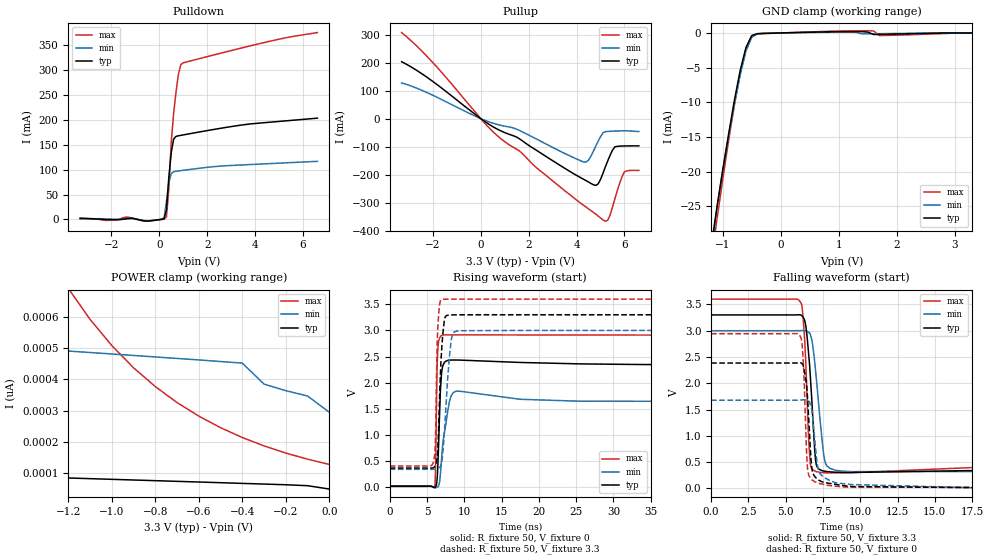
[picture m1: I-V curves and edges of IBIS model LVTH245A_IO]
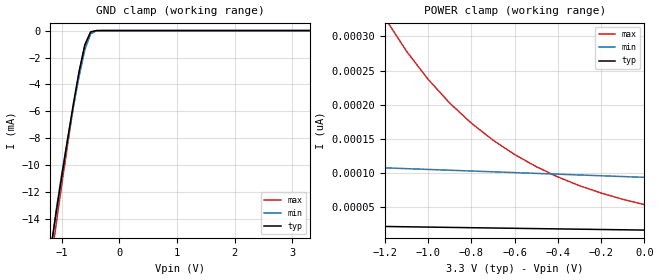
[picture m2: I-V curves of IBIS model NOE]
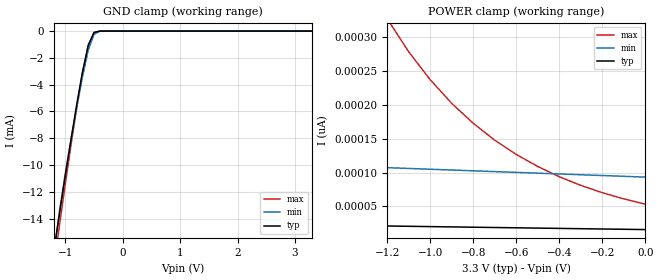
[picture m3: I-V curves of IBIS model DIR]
|   TEXAS INSTRUMENTS INCORPORATED
|   Standard Linear and Logic
|   IBIS Model of SN54LVTH245A
|   3.3V ABT OCTAL BUS  TRANSCEIVERS WITH 3-STATE OUTPUT
| This file contains package information for the following:
|   CFP 20-pin (W) package as [Component] LVTH245A_W
[IBIS Ver]   2.1
[Comment char]   |_char
[File Name]   sn54lvth245aw.ibs
[File Rev]   1.0
[Date]   06-13-2000
[Source]   Data created from HSPICE simulations at TI ,SLL.
[Notes]   The following is an IBIS list for LVTH245A.
   - All test data contained in this file are derived from hspice
   (tm) simulations.
   - - This file may be incomplete or may not be fully compliant
   with the IBIS specification. It will be replaced with a
   version that is IBIS Revision 3.2 compliant and is complete
   and accurate. Please email all questions and comments to
   sllibis@ti.com.
|   -For Questions or Comments please mailto:sllibis@ti.com
|  [Disclaimer]
|*   Property of Texas Instruments Incorporated.  Unauthorized   *
|*   reproduction and/or distribution is strictly prohibited.   *
|*   This product is protected under copyright law.   *
|*   Created 1995, (C) Copyright 1995, Texas Instruments Inc.,   *
|*   All Rights Reserved   *
|*   UNLESS THERE IS A SIGNED, WRITTEN AGREEMENT TO THE   *
|*   CONTRARY, TEXAS INSTRUMENTS ("TI") IS PROVIDING THE SPICE   *
|*   MODELS "AS IS" AND WITHOUT ANY WARRANTY, EXPRESSED OR   *
|*   IMPLIED.  TI assumes no liability for:   *
|*   1) the accuracy of the IBIS models provided to your   *
|*   company;   *
|*   2) the proper functioning of these IBIS models in your   *
|*   design or for any resulting applications; or   *
|*   3) infringement of patents, copyrights or intellectual   *
|*   property rights resulting from your use of these   *
|*   IBIS models.   *
|*   TI provides IBIS Models as a service to our customers.   *
|*   You and your company shall not distribute, sell or give   *
|*   these models to anyone else without prior written   *
|*   permission from TI.   *
|*   TI reserves the right to make changes to our products or   *
|*   to discontinue any semiconductor product or service   *
|*   without notice, and advises our customers to obtain the   *
|*   latest version of relevant information to verify, before   *
|*   placing orders, that the information being relied on is   *
|*   current.   *
|*   Please be aware that your receipt and use of the IBIS   *
|*   information provided shall serve as acceptance of these   *
|*   terms and conditions.  If you do not accept these terms,   *
|*   you should return or destroy the IBIS models and any   *
|*   other accompanying information immediately.   *
[Component]   LVTH245A_W
[manufacturer]   Texas   Instruments,   Inc.
[Package]
|   typ   min   max
R_pkg   0.134   0.093   0.180
L_pkg   6.136e-9   4.282e-9   8.371e-9
C_pkg   1.657e-12   1.224e-12   2.253e-12
[Pin]   signal_name  model_name   R_pin   L_pin   C_pin
1   DIR   DIR   0.161   8.173e-9   2.244e-12
2   A1   LVTH245A_IO   0.163   7.152e-9   2.034e-12
3   A2   LVTH245A_IO   0.154   6.346e-9   1.604e-12
4   A3   LVTH245A_IO   0.093   4.737e-9   1.272e-12
5   A4   LVTH245A_IO   0.097   4.297e-9   1.227e-12
6   A5   LVTH245A_IO   0.096   4.289e-9   1.226e-12
7   A6   LVTH245A_IO   0.093   4.759e-9   1.269e-12
8   A7   LVTH245A_IO   0.143   6.181e-9   1.554e-12
9   A8   LVTH245A_IO   0.164   7.085e-9   1.905e-12
10   GND   GND   0.175   8.294e-9   2.233e-12
11   B8   LVTH245A_IO   0.180   8.371e-9   2.239e-12
12   B7   LVTH245A_IO   0.155   7.195e-9   1.934e-12
13   B6   LVTH245A_IO   0.154   6.339e-9   1.581e-12
14   B5   LVTH245A_IO   0.096   4.872e-9   1.281e-12
15   B4   LVTH245A_IO   0.097   4.338e-9   1.233e-12
16   B3   LVTH245A_IO   0.097   4.282e-9   1.224e-12
17   B2   LVTH245A_IO   0.093   4.726e-9   1.262e-12
18   B1   LVTH245A_IO   0.143   6.164e-9   1.571e-12
19   NOE   NOE   0.159   6.938e-9   2.001e-12
20   VCC   POWER   0.166   8.186e-9   2.253e-12
| Models and submodels in the file (3): LVTH245A_IO (I/O), NOE (Input), DIR (Input)
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|   Model LVTH245A  I/O
[Model]   LVTH245A_IO
|Signals
Model_type  I/O
Polarity   Non-Inverting
Enable   Active-Low
Vinl = 0.8V
Vinh = 2.0V
Vmeas= 1.5V
Cref = 50pf
Rref = 500
Vref = 0V
| variable   typ   min   max
C_comp   9p   NA   NA
[Temperature Range]   50   100   0
[Voltage range]   3.3   3   3.6
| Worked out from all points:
|   slope of the pulldown table from 0 to 0.495 V, typ, clamps not added: 3.74 ohm
|   slope of the pullup table from 0 to 0.495 V, typ, clamps not added: 17.5 ohm
|   GND clamp passes 1 mA (typ) near -0.54 V on its own axis
|   rising waveform, R_fixture 50, V_fixture 0: 20-80 % time 334ps typ, 787ps min, 187ps max; typ from 0.015 V to 2.34 V
|   falling waveform, R_fixture 50, V_fixture 3.3: 20-80 % time 407ps typ, 539ps min, 282ps max; typ from 3.3 V to 0.361 V
|   rising waveform, R_fixture 50, V_fixture 3.3: 20-80 % time 487ps typ, 748ps min, 267ps max; typ from 0.363 V to 3.3 V
|   falling waveform, R_fixture 50, V_fixture 0: 20-80 % time 301ps typ, 395ps min, 226ps max; typ from 2.38 V to 0.015 V
|Process range|   weak   strong
[Pullup]
|   50C:3.3V:   100C:3V:weak   0C:3.6V:strong
|   Voltage   I(typ)   I(min)   I(max)
-3.3V     203.1mA    127.3mA    307.1mA
-2V       132.7mA    83.36mA    200.3mA
500mV     -28.53mA   -16.16mA   -45.85mA
1.5V      -66.22mA   -37.93mA   -109.4mA
4.3V      -217.1mA   -155.1mA   -310.2mA
4.5V      -226.5mA   -148.4mA   -322.3mA
4.8V      -238.8mA   -98.67mA   -341.2mA
5.2V      -173.2mA   -46.97mA   -366.8mA
5.4V      -131.2mA   -45.38mA   -344.5mA
5.6V      -101.1mA   -44.62mA   -286.1mA
6V        -97.81mA   -43.69mA   -190.1mA
6.6V      -97.49mA   -46.24mA   -185.2mA
[Pulldown]
|   50C:3.3V:   100C:3V:weak   0C:3.6V:strong
|   Voltage   I(typ)   I(min)   I(max)
-3.3V     2.372mA    1.132mA    2.209mA
100mV     237.9uA    350.5uA    100.7uA
200mV     1.235mA    3.577mA    847.1uA
300mV     19.22mA    35.89mA    5.175mA
400mV     84.98mA    73.59mA    61.36mA
500mV     134.2mA    92.25mA    155.8mA
600mV     161.2mA    95.76mA    213.1mA
700mV     166.6mA    96.57mA    256.3mA
800mV     167.8mA    97.24mA    291.1mA
900mV     168.7mA    97.89mA    310.7mA
3.6V      190.4mA    109.7mA    345.9mA
6.6V      203.2mA    116.6mA    374.8mA
[GND Clamp]
|   50C:3.3V:   100C:3V:weak   0C:3.6V:strong
|   Voltage   I(typ)   I(min)   I(max)
-3.3V     -626.4mA   -591.3mA   -680.6mA
-1.2V     -30.81mA   -32.23mA   -32.92mA
-1.1V     -25.16mA   -25.2mA    -26.88mA
-900mV    -14.66mA   -14.89mA   -15.59mA
-700mV    -5.437mA   -6.128mA   -5.899mA
-600mV    -2.11mA    -2.619mA   -2.27mA
-500mV    -382.9uA   -616.2uA   -399.1uA
-200mV    -45.64uA   -31.21uA   -65.88uA
1.4V      189.6uA    -126.3uA   320.1uA
1.6V      -220.2uA   -114.9uA   285.4uA
1.7V      -211.2uA   -105.7uA   -367.5uA
3.3V      49.01pA    384.5pA    -3.178nA
[POWER Clamp]
|   50C:3.3V:   100C:3V:weak   0C:3.6V:strong
|   Voltage   I(typ)   I(min)   I(max)
-3.3V     132.6pA    589.3pA    21.93nA
-1.2V     84.38pA    490.2pA    690.3pA
-1.1V     82.21pA    485.5pA    591.4pA
-1V       80.06pA    480.8pA    507.7pA
-900mV    77.9pA     476.1pA    436.7pA
-800mV    75.76pA    471.3pA    376.5pA
-700mV    73.62pA    466.6pA    325.5pA
-600mV    71.47pA    461.9pA    282.1pA
-400mV    67.05pA    451.6pA    213.8pA
-300mV    64.88pA    384.5pA    186.9pA
-100mV    59.71pA    346.4pA    144.5pA
0V        49.01pA    294.5pA    127.6pA
[ramp]
| variable   typ   min   max
dV/dt_r   1.4680E+00/3.6232E-10  1.1128E+00/9.3641E-10  1.7543E+00/1.8433E-10
dV/dt_f   1.8000E+00/4.1355E-10  1.6130E+00/5.4301E-10  1.9843E+00/2.8338E-10
[Rising Waveform]
R_fixture = 50
V_fixture = 0
V_fixture_min =0
V_fixture_max = 0
L_fixture = 0nH
C_fixture = 0pF
|   50C:3.3V:   100C:3V:weak   0C:3.6V:strong
|   Time   V(typ)   V(min)   V(max)
0s        14.92mV    10.12mV    20.87mV
6ns       -13.42mV   -12.8mV    854.9uV
6.15ns    5.5mV      -16.5mV    391.4mV
6.35ns    142.1mV    -4.054mV   2.291V
6.45ns    401.6mV    5.473mV    2.651V
6.8ns     1.861V     259.6mV    2.882V
7ns       2.234V     643.7mV    2.906V
8ns       2.43V      1.632V     2.915V
8.95ns    2.433V     1.834V     2.915V
50ns      2.338V     1.642V     2.91V
[Falling Waveform]
R_fixture = 50
V_fixture = 3.3
V_fixture_min = 3
V_fixture_max = 3.6
L_fixture = 0nH
C_fixture = 0pF
|   50C:3.3V:   100C:3V:weak   0C:3.6V:strong
|   Time   V(typ)   V(min)   V(max)
0s        3.3V       3V         3.6V
6ns       3.301V     3.002V     3.538V
6.25ns    3.211V     3.003V     2.92V
6.55ns    2.514V     2.966V     866.7mV
6.65ns    2.131V     2.932V     470.4mV
6.95ns    709mV      2.392V     332.9mV
7.1ns     412mV      1.946V     316mV
7.65ns    325.7mV    491mV      296mV
8.45ns    307.3mV    340.4mV    295.3mV
50ns      360.6mV    337.2mV    400.9mV
[Rising Waveform]
R_fixture = 50
V_fixture = 3.3
V_fixture_min = 3
V_fixture_max = 3.6
L_fixture = 0nH
C_fixture = 0pF
|   50C:3.3V:   100C:3V:weak   0C:3.6V:strong
|   Time   V(typ)   V(min)   V(max)
0s        362.6mV    338.1mV    402.5mV
5.8ns     365mV      337mV      452.6mV
6.1ns     412.6mV    342.5mV    784.8mV
6.35ns    554.2mV    352.3mV    2.684V
6.45ns    747.6mV    357.9mV    3.071V
7ns       2.717V     513.9mV    3.592V
7.4ns     3.242V     1.211V     3.598V
8.2ns     3.297V     2.764V     3.6V
8.9ns     3.299V     2.985V     3.6V
50ns      3.3V       3V         3.6V
[Falling Waveform]
R_fixture = 50
V_fixture = 0
V_fixture_min = 0
V_fixture_max = 0
L_fixture = 0nH
C_fixture = 0pF
|   50C:3.3V:   100C:3V:weak   0C:3.6V:strong
|   Time   V(typ)   V(min)   V(max)
0s        2.385V     1.677V     2.944V
5.9ns     2.39V      1.679V     2.925V
6.15ns    2.355V     1.686V     2.548V
6.4ns     1.964V     1.682V     676.4mV
6.5ns     1.539V     1.665V     303.7mV
6.7ns     535.9mV    1.547V     180.4mV
6.8ns     311mV      1.356V     155.8mV
7.15ns    172.8mV    402.9mV    107.5mV
7.75ns    105.2mV    180.7mV    62.15mV
50ns      14.94mV    10.83mV    20.95mV
|   LVTH245A NOE
[Model]   NOE
| Signals
Model_type  Input
Polarity   Non-Inverting
Vinl = 0.8V
Vinh = 2.0V
| variable   typ   min   max
C_comp   4p   NA   NA
[Temperature Range]   50   100   0
[Voltage range]   3.3   3   3.6
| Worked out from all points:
|   GND clamp passes 1 mA (typ) near -0.59 V on its own axis
|Process range|   weak   strong
[GND Clamp]
|   50C:3.3V:   100C:3V:weak   0C:3.6V:strong
|   Voltage   I(typ)   I(min)   I(max)
-3.3V     -124.6mA   -123.1mA   -127.8mA
-1.2V     -16.41mA   -16.78mA   -17.55mA
-1.1V     -13.57mA   -13.4mA    -14.44mA
-1V       -10.8mA    -10.61mA   -11.42mA
-900mV    -8.089mA   -8.088mA   -8.489mA
-800mV    -5.459mA   -5.679mA   -5.686mA
-700mV    -3.041mA   -3.403mA   -3.115mA
-600mV    -1.069mA   -1.419mA   -1.046mA
-500mV    -98.9uA    -244.7uA   -120.4uA
-400mV    -3.202uA   -14.58uA   -1.224uA
-300mV    -89.54nA   -666.4nA   -17.62nA
3.3V      15.84pA    96.72pA    36.16pA
[POWER Clamp]
|   50C:3.3V:   100C:3V:weak   0C:3.6V:strong
|   Voltage   I(typ)   I(min)   I(max)
-3.3V     32.07pA    131.6pA    10.93nA
-1.2V     21.13pA    107.2pA    327.1pA
-1.1V     20.67pA    106pA      278.2pA
-1V       20.22pA    104.9pA    237pA
-900mV    19.77pA    103.7pA    202.1pA
-800mV    19.32pA    102.5pA    172.7pA
-700mV    18.88pA    101.4pA    147.8pA
-600mV    18.44pA    100.2pA    126.7pA
-500mV    18pA       99.04pA    108.9pA
-400mV    17.56pA    97.88pA    93.79pA
-200mV    16.7pA     95.56pA    70.2pA
0V        15.84pA    93.24pA    53.23pA
|   LVTH245A DIR
[Model]   DIR
| Signals
Model_type  Input
Vinl = 0.8V
Vinh = 2.0V
| variable   typ   min   max
C_comp   4p   NA   NA
[Temperature Range]   50   100   0
[Voltage range]   3.3   3   3.6
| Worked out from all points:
|   GND clamp passes 1 mA (typ) near -0.59 V on its own axis
|Process range|   weak   strong
[GND Clamp]
|   50C:3.3V:   100C:3V:weak   0C:3.6V:strong
|   Voltage   I(typ)   I(min)   I(max)
-3.3V     -124.6mA   -123.1mA   -127.8mA
-1.2V     -16.41mA   -16.78mA   -17.55mA
-1.1V     -13.57mA   -13.4mA    -14.44mA
-1V       -10.8mA    -10.61mA   -11.42mA
-900mV    -8.089mA   -8.088mA   -8.489mA
-800mV    -5.459mA   -5.679mA   -5.686mA
-700mV    -3.041mA   -3.403mA   -3.115mA
-600mV    -1.069mA   -1.419mA   -1.046mA
-500mV    -98.9uA    -244.7uA   -120.4uA
-400mV    -3.202uA   -14.58uA   -1.224uA
-300mV    -89.54nA   -666.4nA   -17.62nA
3.3V      15.84pA    96.72pA    36.16pA
[POWER Clamp]
|   50C:3.3V:   100C:3V:weak   0C:3.6V:strong
|   Voltage   I(typ)   I(min)   I(max)
-3.3V     32.07pA    131.6pA    10.93nA
-1.2V     21.13pA    107.2pA    327.1pA
-1.1V     20.67pA    106pA      278.2pA
-1V       20.22pA    104.9pA    237pA
-900mV    19.77pA    103.7pA    202.1pA
-800mV    19.32pA    102.5pA    172.7pA
-700mV    18.88pA    101.4pA    147.8pA
-600mV    18.44pA    100.2pA    126.7pA
-500mV    18pA       99.04pA    108.9pA
-400mV    17.56pA    97.88pA    93.79pA
-200mV    16.7pA     95.56pA    70.2pA
0V        15.84pA    93.24pA    53.23pA
